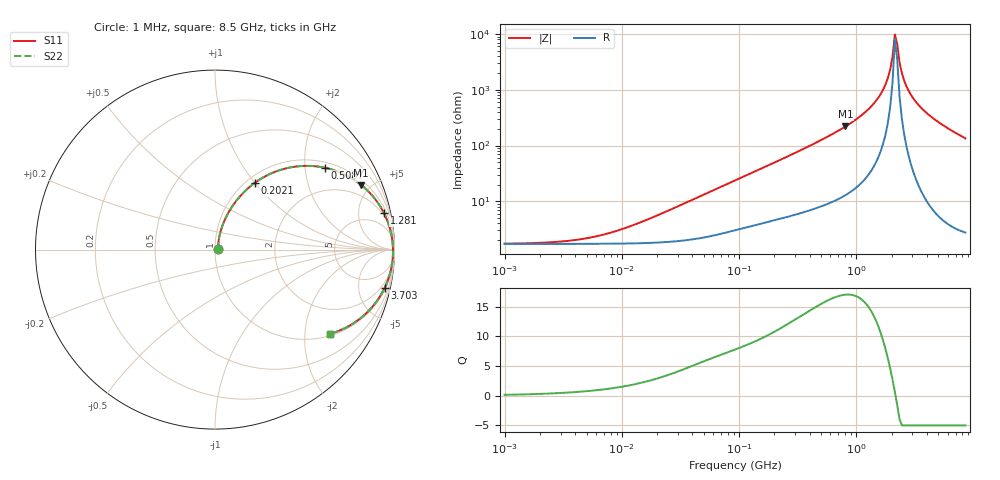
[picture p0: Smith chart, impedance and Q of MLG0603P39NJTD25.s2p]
! S-Parameter Data Generated by TDK Corporation
! Copyright(C) 2025 TDK Corporation.
! All Rights Reserved.
! TDK P/N: MLG0603P39NJTD25 (SMD / SMT Inductor (Coil))
! Property: L=39nH at 300MHz
! Size(LxWxT): 0.6x0.3x0.3mm
! Model Type: s2p (Touchstone File Format Version 1.0)
! Frequency: DC=Yes Start=1MHz Stop=8500MHz 198points Log-sweep
! Model Generated on Feb. 6, 2025
! Terms and conditions regarding TDK Simulation Models:
! 1)This simulation model is being provided solely for informational
!  purposes. Please refer to the specifications of the products in
!  terms of detailed characteristics of such products.
! 2)In no event shall TDK Corporation of any of its subsidiaries be
!  liable for any loss or damage arising, directly or indirectly,
!  from any information contained in this simulation model, including,
!  but not limited to loss or damages arising from any inaccuracies,
!  omissions or errors in connection with such information.
! 3)Any and all copyrights on this simulation model are owned by
!  TDK Corporation.  Duplication or redistribution of this simulation
!  model without prior written permission from TDK Corporation
!  is prohibited.
! 4)This simulation model is subject to any modification or change
!  without any prior notice.
! 5)Neither TDK Corporation nor any of its subsidiaries shall make any
!  warranty, express or implied, including but not limited to the
!  correctness, implied warranties of merchantability and fitness for
!  a particular purpose with respect to this simulation models.
! 6)The use of this simulation model shall be deemed to have consented
!  to the terms and conditions hereof.
! Port Assignments:
!  1 ---@@@--- 2
! Applicable Conditions:
!  Temperature = 25 degC
!  DC Bias Current = 0 A
!  Small Signal Operation
# Hz S MA R 50
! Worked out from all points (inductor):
!   197 points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, 1 MHz to 8.5 GHz, reference 50 ohm
!   read as one part in series: L = 41.8 nH near 21.05 MHz
!   highest Q = 17 at 807.2 MHz (marker M1), where L = 43.3 nH
!   self-resonance near 2.128 GHz
!   S11 on the Smith chart (normalised r, x): 1 MHz: 1.03, +0.01; 202.1 MHz: 1.09, +1.00; 508.7 MHz: 1.16, +2.55; 1.281 GHz: 1.62, +9.15; 3.703 GHz: 1.26, -8.76; 8.5 GHz: 1.06, -2.69
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1000000  0.01711 8.6  0.9831 -0.1  0.9831 -0.1  0.01711 8.6
4587603  0.02073 34.4  0.983 -0.7  0.983 -0.7  0.02073 34.4
9168677  0.0293 52.9  0.9826 -1.4  0.9826 -1.4  0.0293 52.9
2.10461e7  0.05722 68.6  0.9806 -3.1  0.9806 -3.1  0.05722 68.6
9.219544e7  0.2235 69.9  0.9466 -12.8  0.9466 -12.8  0.2235 69.9
2.020814e8  0.4314 59.3  0.8634 -25.4  0.8634 -25.4  0.4314 59.3
4.229561e8  0.7 41.8  0.668 -44.3  0.668 -44.3  0.7 41.8
5.087302e8  0.7637 36.7  0.5984 -49.6  0.5984 -49.6  0.7637 36.7
8.071757e8  0.8907 23.9  0.4053 -62.8  0.4053 -62.8  0.8907 23.9
1.280704e9  0.9637 12.1  0.21 -74.0  0.21 -74.0  0.9637 12.1
1.689417e9  0.9848 5.6  0.09796 -78.3  0.09796 -78.3  0.9848 5.6
1.852819e9  0.9886 3.5  0.06135 -77.6  0.06135 -77.6  0.9886 3.5
1.940355e9  0.9899 2.4  0.04323 -75.3  0.04323 -75.3  0.9899 2.4
2.032026e9  0.9909 1.4  0.02547 -68.4  0.02547 -68.4  0.9909 1.4
2.128028e9  0.9915 0.3  0.01011 -33.1  0.01011 -33.1  0.9915 0.3
2.228565e9  0.9918 -0.7  0.01516 56.8  0.01516 56.8  0.9918 -0.7
2.333852e9  0.9917 -1.8  0.03217 74.1  0.03217 74.1  0.9917 -1.8
2.559585e9  0.9903 -3.9  0.0686 79.9  0.0686 79.9  0.9903 -3.9
2.939772e9  0.9854 -7.1  0.1246 79.7  0.1246 79.7  0.9854 -7.1
3.703002e9  0.9687 -12.8  0.2211 75.5  0.2211 75.5  0.9687 -12.8
5.357206e9  0.9157 -22.6  0.384 66.3  0.384 66.3  0.9157 -22.6
8.5e9  0.7947 -36.2  0.591 52.6  0.591 52.6  0.7947 -36.2
